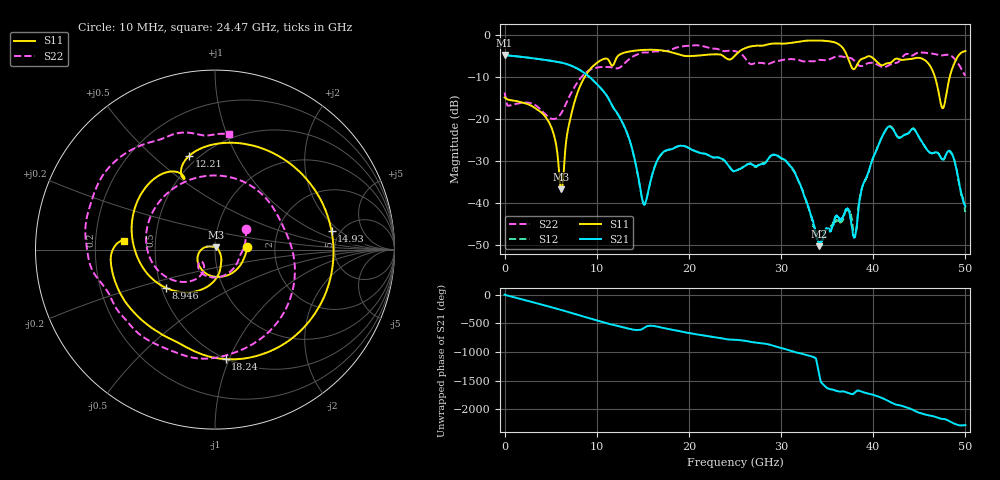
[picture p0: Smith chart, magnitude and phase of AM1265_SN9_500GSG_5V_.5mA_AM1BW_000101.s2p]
!Keysight Technologies,N5245B,MY58422270,A.16.20.02
!Date: Thursday, March 05, 2026 00:29:09
!Correction: S11(C  2-Port  )
!S21(C  2-Port  )
!S12(C  2-Port  )
!S22(C  2-Port  )
!S2P File: Measurements: S11, S21, S12, S22:
# Hz S  dB  R 50
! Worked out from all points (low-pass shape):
!   3201 points, 10 MHz to 50 GHz, reference 50 ohm
!   highest |S21| = -4.79 dB at 10 MHz (marker M1); lowest = -50.4 dB at 34.16 GHz (marker M2)
!   |S21| within 3 dB of the highest: start of sweep to 7.668 GHz
!   lowest |S11| = -36.8 dB at 6.165 GHz (marker M3), VSWR 1.03, Z = 50.6 + j1.32 ohm
!   |S11| at or under -10 dB: start of sweep to 8.714 GHz; 46.69 GHz to 48.3 GHz (1.613 GHz wide, 3.4 % of centre)
!   |S22| runs from -20.1 to -2.5 dB; largest |S21 - S12| = 0.0098
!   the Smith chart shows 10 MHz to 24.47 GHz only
!   S11 on the Smith chart (normalised r, x): 10 MHz: 1.43, +0.04; 8.946 GHz: 0.53, -0.26; 12.21 GHz: 0.45, +0.66; 14.93 GHz: 4.27, +1.53; 18.24 GHz: 0.50, -0.97; 24.47 GHz: 0.33, +0.04
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1e7  -14.93 4.7  -4.79 3.4  -4.75 2.5  -13.75 34.1
2.306416e9  -16.37 -89.4  -5.39 -98.4  -5.39 -98.4  -16.15 -98.2
4.196662e9  -18.93 -149.8  -5.92 -179.0  -5.92 -179.0  -18.45 -139.9
6.165019e9  -36.78 63.8  -6.64 93.4  -6.64 93.4  -18.65 -121.2
8.352081e9  -11.50 -117.6  -8.65 -10.3  -8.64 -10.2  -10.06 -151.5
8.945712e9  -9.20 -142.1  -9.58 -38.5  -9.57 -38.5  -8.81 -171.0
1.096093e10  -5.67 134.8  -14.10 -131.9  -14.09 -131.9  -7.67 101.9
1.221068e10  -5.32 105.3  -18.64 177.7  -18.63 177.6  -8.01 29.0
1.492889e10  -3.64 8.9  -39.14 119.2  -39.16 119.2  -4.26 -96.9
1.667854e10  -3.65 -43.8  -29.48 159.3  -29.51 159.3  -3.98 -141.2
1.824073e10  -4.24 -84.5  -27.19 107.8  -27.11 107.7  -3.42 -166.4
2.447386e10  -5.89 174.6  -31.72 -64.5  -31.62 -64.6  -3.77 83.2
2.5005e10  -4.97 173.7  -32.45 -66.4  -32.52 -66.5  -3.90 70.9
2.95041e10  -2.06 95.9  -28.70 172.5  -28.64 172.0  -6.28 -19.4
3.334708e10  -1.39 35.6  -43.56 2.7  -44.16 3.6  -6.33 -127.7
3.415942e10  -1.37 21.5  -50.36 32.6  -50.07 -176.2  -6.00 -144.4
3.670578e10  -3.17 -31.6  -43.36 111.6  -43.95 106.8  -5.22 165.2
3.80024e10  -8.06 -26.5  -48.17 89.9  -47.95 132.2  -6.35 139.5
4.167354e10  -6.77 -54.2  -21.90 -59.8  -21.88 -59.1  -7.30 116.4
4.511035e10  -5.56 -102.3  -24.91 91.1  -24.97 91.7  -4.22 75.9
4.770358e10  -16.78 69.9  -29.48 -12.5  -29.58 -11.4  -4.83 40.0
5e10  -3.88 -73.0  -40.87 -119.7  -42.15 -140.6  -9.73 2.9
